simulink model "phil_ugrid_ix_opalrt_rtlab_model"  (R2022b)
settings: Solver=ode3  StartTime=0.0  StopTime=inf  FixedStep=Ts  RelTol=1e-3
PostLoadFcn:
  | phil_ugrid_ix_opalrt_rtlab_param;
InitFcn:
  | phil_ugrid_ix_opalrt_rtlab_param;
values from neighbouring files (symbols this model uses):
  GridFreq = 50    [phil_ugrid_ix_opalrt_rtlab_param.m]
  KiIg = 1/Ti2*1/5    (= 165)    [phil_ugrid_ix_opalrt_rtlab_param.m]
  KpIg = Tn2/Ti2*1/3    (= 18.3333333333)    [phil_ugrid_ix_opalrt_rtlab_param.m]
  Lg = 2.2e-3    (= 0.0022)    [phil_ugrid_ix_opalrt_rtlab_param.m]
  PLL_BW = 30    [phil_ugrid_ix_opalrt_rtlab_param.m]
  PLL_FREQ = 50    [phil_ugrid_ix_opalrt_rtlab_param.m]
  PLL_zeta = 1/sqrt(2)    [phil_ugrid_ix_opalrt_rtlab_param.m]
undefined symbols (not defined in the file or in its folder): af15, arm1_g1, Boost2lvl_SFun, boost_I, boost_V, C, c62c8459, DB, DiscIntNeverNeededParam, EFPGASIMConfig, eHSBuildReport, eHSx64_Gen4_Machines_IOConfig1, EX, fault_sw, LABv2024, logs, matlab, Min, models, ns, OPAL, phil_ugrid_ix_opalrt_rtlab, phil_ugrid_ix_opalrt_rtlab_ehs, phil_ugrid_ix_opalrt_rtlab_model, phil_ugrid_ix_opalrt_rtlab_param, RT, Step, TE0741_4, Time, Users, v1, vin, vsrc1, vsrc2, vsrc3
libraries: simulink x6, opal_lib x3, rtlab x2, slpidlib x2, rtio_opalrt_common x1, ehsSchematicEditorSourceLib x1

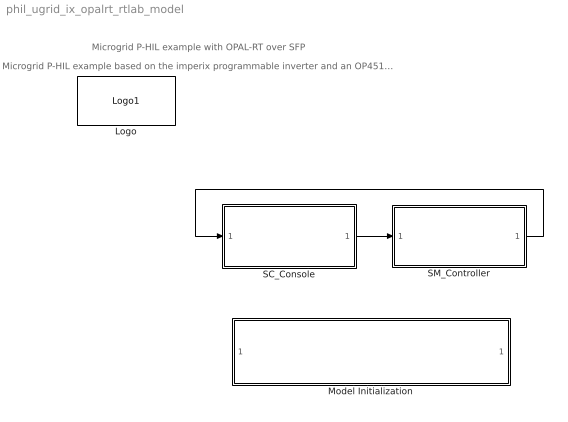
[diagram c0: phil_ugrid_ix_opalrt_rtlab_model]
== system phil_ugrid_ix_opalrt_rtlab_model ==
  note: Microgrid P-HIL example based on the imperix programmable inverter and an OP4510 from OPAL-RT.
  note: Microgrid P-HIL example with OPAL-RT over SFP
  Logo : opal_lib/Logo1  vide=[]
  Model Initialization : Subsystem  mask(Model Functions){InitFcnX=phil_ugrid_ix_opalrt_rtlab_param;, prel=off, posl=on, inif=on, strf=off}
      mask prompts: InitFcnX "Initialisation"; prel "Preload Function"; posl "PostLoad Function"; inif "InitFcn"; strf "StartFcn"
      mask init:
      | currentBlock = gcb;
      | root = bdroot(currentBlock);
      | 
      | if ~strcmp(get_param(root,'BlockDiagramType'),'library')
      |     if prel==1
      |         set_param(root, 'PreLoadFcn', InitFcnX);
      |     else
      |         set_param(root, 'PreLoadFcn', '');
      |     end
      |     if inif==1
      |         set_param(root, 'InitFcn', InitFcnX);
      |     else
      |         set_param(root, 'InitFcn', '');
      |     end
      |     if strf==1
      |         set_param(root, 'StartFcn', InitFcnX);
      |     else
      |         set_param(root, 'StartFcn', '');
      |     end
      |     if posl==1
      |         set_param(root, 'PostLoadFcn', InitFcnX);
      |     else
      |         set_param(root, 'PostLoadFcn', '');
      |     end
      | end
      | 
      | pos = get_param(currentBlock, 'Position');
      | width = pos(3) - pos(1); height = pos(4) - pos(2);
      | txt = [ upper(root) '\n' '- InitFcn. . . . . '  get_param(root, 'InitFcn') ];
  SC_Console : Subsystem
  SM_Controller : Subsystem
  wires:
  SC_Console/1(to_eHS) -> SM_Controller/1(to_eHS)
  SM_Controller/1(from_eHS) -> SC_Console/1(from_eHS)

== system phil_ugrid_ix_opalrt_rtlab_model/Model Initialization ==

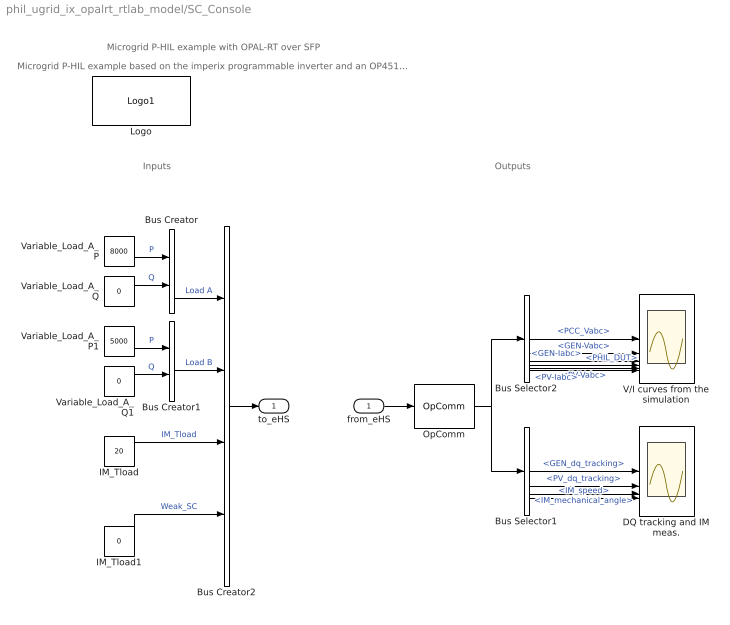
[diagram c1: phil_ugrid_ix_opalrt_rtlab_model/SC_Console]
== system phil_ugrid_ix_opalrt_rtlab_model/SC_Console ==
  note: Inputs
  note: Outputs
  note: Microgrid P-HIL example based on the imperix programmable inverter and an OP4510 from OPAL-RT.
  note: Microgrid P-HIL example with OPAL-RT over SFP
  from_eHS : Inport  OutDataTypeStr=double
  Bus Creator : BusCreator  Inputs=2
  Bus Creator1 : BusCreator  Inputs=2
  Bus Creator2 : BusCreator  Inputs=4
  Bus Selector1 : BusSelector  OutputSignals=signal2.GEN_dq_tracking,signal2.PV_dq_tracking,signal1.IM.IM_mechanical_angle,signal1.IM.IM_speed
  Bus Selector2 : BusSelector  OutputSignals=signal1.PCC_Vabc,signal1.GEN-Vabc,signal1.GEN-Iabc,signal1.PHIL_DUT,signal1.PV-Vabc,signal1.PV-Iabc
  DQ tracking and IM meas. : Scope  NumInputPorts=4
  IM_Tload : Constant  Value=20
  IM_Tload1 : Constant  Value=0
  Logo : opal_lib/Logo1  vide=[]
  OpComm : rtlab/OpComm  nbport=1  groupe_acq=1  subsys_rate=0  st=0  Synchronization=off  Interpolation=off  Threshold=1.0  Missed_Data=off  Sim_Time=off  Samples=off  dynSigOut=off  from_console=0  warning_done=off  writeOpCommFile=off
  V/I curves from the simulation : Scope  NumInputPorts=6
  Variable_Load_A_P : Constant  Value=8000
  Variable_Load_A_P1 : Constant  Value=5000
  Variable_Load_A_Q : Constant  Value=0
  Variable_Load_A_Q1 : Constant  Value=0
  to_eHS : Outport  VectorParamsAs1DForOutWhenUnconnected=off
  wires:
  from_eHS/1 -> OpComm/1
  Bus Creator2/1 -> to_eHS/1
  OpComm/1 -> Bus Selector1/1, Bus Selector2/1
  Variable_Load_A_P/1 -> Bus Creator/1  "P"
  Variable_Load_A_Q/1 -> Bus Creator/2  "Q"
  Variable_Load_A_P1/1 -> Bus Creator1/1  "P"
  Variable_Load_A_Q1/1 -> Bus Creator1/2  "Q"
  Bus Creator/1 -> Bus Creator2/1  "Load A"
  Bus Creator1/1 -> Bus Creator2/2  "Load B"
  IM_Tload/1 -> Bus Creator2/3  "IM_Tload"
  Bus Selector2/1 -> V/I curves from the simulation/1  "<PCC_Vabc>"
  Bus Selector2/2 -> V/I curves from the simulation/2  "<GEN-Vabc>"
  Bus Selector2/3 -> V/I curves from the simulation/3  "<GEN-Iabc>"
  Bus Selector2/4 -> V/I curves from the simulation/4  "<PHIL_DUT>"
  Bus Selector2/5 -> V/I curves from the simulation/5  "<PV-Vabc>"
  Bus Selector2/6 -> V/I curves from the simulation/6  "<PV-Iabc>"
  Bus Selector1/1 -> DQ tracking and IM meas./1  "<GEN_dq_tracking>"
  Bus Selector1/2 -> DQ tracking and IM meas./2  "<PV_dq_tracking>"
  Bus Selector1/3 -> DQ tracking and IM meas./3  "<IM_mechanical_angle>"
  Bus Selector1/4 -> DQ tracking and IM meas./4  "<IM_speed>"
  IM_Tload1/1 -> Bus Creator2/4  "Weak_SC"

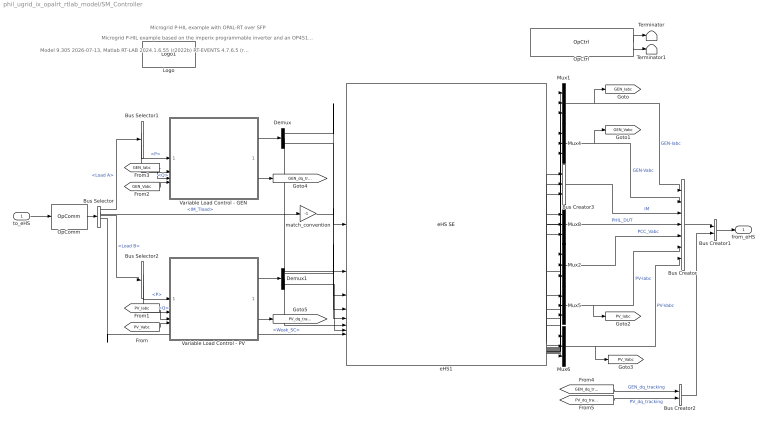
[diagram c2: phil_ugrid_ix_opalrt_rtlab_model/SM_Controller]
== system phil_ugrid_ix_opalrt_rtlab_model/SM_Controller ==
  note: Model 9.305 2026-07-13, Matlab RT-LAB 2024.1.6.55 (r2022b) RT-EVENTS 4.7.6.5 (r2022b.x) eFPGAsim () &copy; 2026 Opal-RT Technologies Inc.
  note: Microgrid P-HIL example with OPAL-RT over SFP
  note: Microgrid P-HIL example based on the imperix programmable inverter and an OP4510 from OPAL-RT.
  to_eHS : Inport
  Bus Creator : BusCreator  Inputs=7
  Bus Creator1 : BusCreator  Inputs=2
  Bus Creator2 : BusCreator  Inputs=2
  Bus Creator3 : BusCreator  Inputs=3
  Bus Selector : BusSelector  OutputSignals=Load A,IM_Tload,Load B,Weak_SC
  Bus Selector1 : BusSelector  OutputSignals=P,Q
  Bus Selector2 : BusSelector  OutputSignals=P,Q
  Demux : Demux  Outputs=3
  Demux1 : Demux  Outputs=3
  Logo : opal_lib/Logo1  vide=[]
  Mux{1..2,4..6,8} (6 alike) : Mux  Inputs=3
  OpComm : rtlab/OpComm  nbport=1  groupe_acq=1  subsys_rate=0  st=0  Synchronization=on  Interpolation=on  Threshold=1.0  Missed_Data=off  Sim_Time=off  Samples=off  dynSigOut=off  from_console=1  warning_done=off  writeOpCommFile=off
  OpCtrl : rtio_opalrt_common/OpCtrl  CtrlName='OpCtrl'  boardid=0  BitstreamFilename=TE0741_4-EX-0001-3_11_2_12-eHSx64_Gen4_Machines_IOConfig1-DB-4A.bin  numconfig=-1  mode=Master  externalClock=off  decimRtsi=0  calibIO=off  SampleTime=0  loadinport=-1  BoardType=TE0741  SecondaryPresent=off  sync_type=Audio  scope_enable=off  fsdFileName=TE0741_4-EX-0001-3_11_2_12-eHSx64_Gen4_Machines_IOConfig1-DB-4A.fsd  mismatch_disable=on
  Terminator : Terminator
  Terminator1 : Terminator
  Variable Load Control - GEN : Subsystem
  Variable Load Control - PV : Subsystem
  eHS1 : ehsSchematicEditorSourceLib/eHS SE  modelName=Boost2lvl_SFun - v1  modelUuid=c62c8459-3f79-48c0-af15-759a73c628dc  modelDisplayName=Boost2lvl_SFun  lastLoadedModelText=Circuit loaded on 09-Oct-2024 14:20:43  lastLoadedModelName=Boost2lvl_SFun - v1  lastLoadedModelUuid=c62c8459-3f79-48c0-af15-759a73c628dc  lastLoadedModelDisplayName=Boost2lvl_SFun - v1  triggerUpdate=off  timeStepInfo=Time Step: 230 ns (Min: 230 ns)  inputPins=arm1_g1,fault_sw,vin,vsrc1,vsrc2,vsrc3  outputPins=2Lvl_Ia,2Lvl_Ib,2Lvl_Ic,2Lvl_Va,2Lvl_Vb,2Lvl_Vc,boost_I,boost_V  loadPassed=1  firmwareName=TE0741_4-EX-0001-3_11_2_12-eHSx64_Gen4_Machines_IOConfig1-DB-4A.bin  driverType=SFUN  ehsEffectiveLicense=x128  migrated=on  opCtrlName='OpCtrl'  autoConfigureFirmware=on  ehsFileName=phil_ugrid_ix_opalrt_rtlab_ehs.ehs3  buildReportFile=C:\Users\matlab\OPAL-RT\RT-LABv2024.1_Workspace2\phil_ugrid_ix_opalrt_rtlab\models\phil_ugrid_ix_opalrt_rtlab_model\EFPGASIMConfig\logs\phil_ugrid_ix_opalrt_rtlab_ehs\logs\eHSBuildReport.txt  displayBlockInfos=|
      | x32
      | Time Step: 355 ns (Min: 355 ns)
  match_convention : Gain  Gain=-1
  from_eHS : Outport  VectorParamsAs1DForOutWhenUnconnected=off
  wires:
  to_eHS/1 -> OpComm/1
  OpComm/1 -> Bus Selector/1
  OpCtrl/1 -> Terminator/1
  OpCtrl/2 -> Terminator1/1
  Mux2/1 -> Bus Creator/5  "PCC_Vabc"
  Bus Selector1/1 -> Variable Load Control - GEN/1(P)  "<P>"
  Bus Selector1/2 -> Variable Load Control - GEN/2(Q)  "<Q>"
  Bus Selector/1 -> Bus Selector1/1  "<Load A>"
  Variable Load Control - GEN/1(Vabc) -> Demux/1
  Demux/2 -> eHS1/2
  Demux/1 -> eHS1/1
  Demux/3 -> eHS1/3
  Variable Load Control - PV/1(Vabc) -> Demux1/1
  Demux1/2 -> eHS1/6
  Demux1/3 -> eHS1/7
  Bus Selector/3 -> Bus Selector2/1  "<Load B>"
  Bus Selector2/2 -> Variable Load Control - PV/2(Q)  "<Q>"
  Bus Selector2/1 -> Variable Load Control - PV/1(P)  "<P>"
  eHS1/1 -> Mux1/1
  eHS1/2 -> Mux1/2
  eHS1/3 -> Mux1/3
  eHS1/4 -> Mux4/1
  eHS1/5 -> Mux4/2
  eHS1/6 -> Mux4/3
  Mux1/1 -> Bus Creator/1, [GEN_Iabc]  "GEN-Iabc"
  Mux4/1 -> Bus Creator/2, [GEN_Vabc]  "GEN-Vabc"
  Mux5/1 -> Bus Creator/6, [PV_Iabc]  "PV-Iabc"
  Mux6/1 -> Bus Creator/7, [PV_Vabc]  "PV-Vabc"
  [PV_Vabc] -> Variable Load Control - PV/4(vabc)
  [PV_Iabc] -> Variable Load Control - PV/3(iabc)
  [GEN_Vabc] -> Variable Load Control - GEN/4(vabc)
  [GEN_Iabc] -> Variable Load Control - GEN/3(iabc)
  Mux8/1 -> Bus Creator/4  "PHIL_DUT"
  Bus Selector/2 -> match_convention/1  "<IM_Tload>"
  eHS1/10 -> Mux8/1
  eHS1/11 -> Mux8/2
  eHS1/12 -> Mux8/3
  eHS1/13 -> Mux2/1
  eHS1/14 -> Mux2/2
  eHS1/15 -> Mux2/3
  eHS1/16 -> Mux5/1
  eHS1/17 -> Mux5/2
  eHS1/18 -> Mux5/3
  eHS1/19 -> Mux6/1
  eHS1/20 -> Mux6/2
  eHS1/21 -> Mux6/3
  Bus Creator3/1 -> Bus Creator/3  "IM"
  eHS1/7 -> Bus Creator3/1
  eHS1/9 -> Bus Creator3/3
  Bus Creator1/1 -> from_eHS/1
  Bus Creator/1 -> Bus Creator1/1
  Bus Creator2/1 -> Bus Creator1/2
  Variable Load Control - GEN/2(dq_tracking) -> [GEN_dq_tracking]
  [GEN_dq_tracking] -> Bus Creator2/1  "GEN_dq_tracking"
  Variable Load Control - PV/2(dq_tracking) -> [PV_dq_tracking]
  [PV_dq_tracking] -> Bus Creator2/2  "PV_dq_tracking"
  Demux1/1 -> eHS1/5
  eHS1/8 -> Bus Creator3/2
  Bus Selector/4 -> eHS1/8  "<Weak_SC>"
  match_convention/1 -> eHS1/4

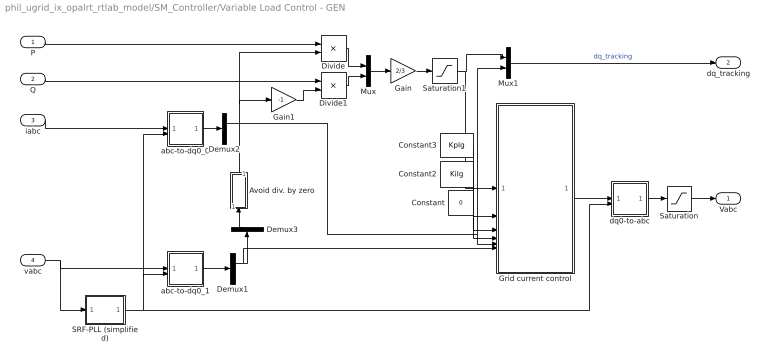
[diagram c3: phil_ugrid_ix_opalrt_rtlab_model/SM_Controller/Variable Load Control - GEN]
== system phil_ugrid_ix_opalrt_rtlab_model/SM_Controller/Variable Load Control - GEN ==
  P : Inport
  Q : Inport  Port=2
  iabc : Inport  Port=3
  vabc : Inport  Port=4
  Avoid div. by zero : Subsystem
  Constant : Constant  Value=0  OutDataTypeStr=double
  Constant2 : Constant  Value=KiIg  OutDataTypeStr=double
  Constant3 : Constant  Value=KpIg  OutDataTypeStr=double
  Demux1 : Demux  Outputs=[2 1]
  Demux2 : Demux  Outputs=[2 1]
  Demux3 : Demux  Outputs=2
  Divide : Product  Inputs=*/
  Divide1 : Product  Inputs=*/
  Gain : Gain  Gain=2/3
  Gain1 : Gain  Gain=-1
  Grid current control : Subsystem
  Mux : Mux  Inputs=2
  Mux1 : Mux  Inputs=2
  SRF-PLL (simplified) : Subsystem
  Saturation : Saturate  UpperLimit=400  LowerLimit=-400
  Saturation1 : Saturate  UpperLimit=50  LowerLimit=-50
  abc-to-dq0_0 : Subsystem
  abc-to-dq0_1 : Subsystem
  dq0-to-abc : Subsystem
  Vabc : Outport
  dq_tracking : Outport  Port=2
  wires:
  Demux3/1 -> Avoid div. by zero/1(In)
  Mux1/1 -> dq_tracking/1  "dq_tracking"
  Divide/1 -> Mux/1
  Divide1/1 -> Mux/2
  Mux/1 -> Gain/1
  Gain1/1 -> Divide1/2
  abc-to-dq0_0/1(dq0) -> Demux2/1
  iabc/1 -> abc-to-dq0_0/1(abc)
  Avoid div. by zero/1(Out) -> Divide/2, Gain1/1
  Gain/1 -> Saturation1/1
  abc-to-dq0_1/1(dq0) -> Demux1/1
  P/1 -> Divide/1
  Q/1 -> Divide1/1
  vabc/1 -> abc-to-dq0_1/1(abc), SRF-PLL (simplified)/1(Vg)
  SRF-PLL (simplified)/1(θ) -> dq0-to-abc/2(wt), abc-to-dq0_0/2(wt), abc-to-dq0_1/2(wt)
  Constant2/1 -> Grid current control/3(Ki_Ig)
  Demux2/1 -> Mux1/2, Grid current control/5(Ig_dq)
  Demux1/1 -> Grid current control/6(Vg_dq), Demux3/1
  Constant/1 -> Grid current control/4(reset)
  Constant3/1 -> Grid current control/2(Kp_Ig)
  Saturation1/1 -> Grid current control/1(Ig_dq_ref), Mux1/1
  dq0-to-abc/1(abc) -> Saturation/1
  Grid current control/1(Eg_dq0*) -> dq0-to-abc/1(dq0)
  Saturation/1 -> Vabc/1

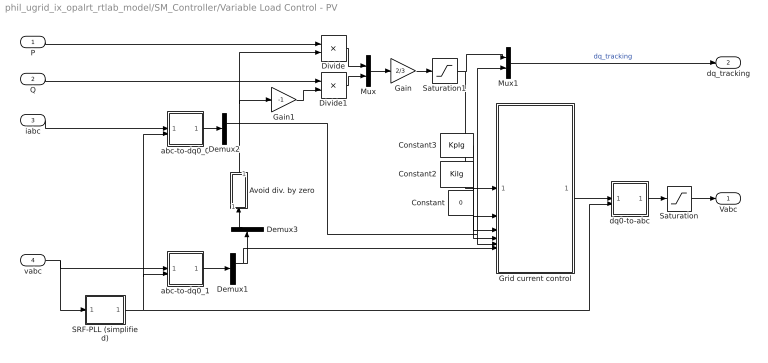
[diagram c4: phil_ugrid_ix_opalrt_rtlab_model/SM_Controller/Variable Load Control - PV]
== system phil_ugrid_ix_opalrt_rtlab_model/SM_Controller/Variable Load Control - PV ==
  P : Inport
  Q : Inport  Port=2
  iabc : Inport  Port=3
  vabc : Inport  Port=4
  Avoid div. by zero : Subsystem
  Constant : Constant  Value=0  OutDataTypeStr=double
  Constant2 : Constant  Value=KiIg  OutDataTypeStr=double
  Constant3 : Constant  Value=KpIg  OutDataTypeStr=double
  Demux1 : Demux  Outputs=[2 1]
  Demux2 : Demux  Outputs=[2 1]
  Demux3 : Demux  Outputs=2
  Divide : Product  Inputs=*/
  Divide1 : Product  Inputs=*/
  Gain : Gain  Gain=2/3
  Gain1 : Gain  Gain=-1
  Grid current control : Subsystem
  Mux : Mux  Inputs=2
  Mux1 : Mux  Inputs=2
  SRF-PLL (simplified) : Subsystem
  Saturation : Saturate  UpperLimit=400  LowerLimit=-400
  Saturation1 : Saturate  UpperLimit=50  LowerLimit=-50
  abc-to-dq0_0 : Subsystem
  abc-to-dq0_1 : Subsystem
  dq0-to-abc : Subsystem
  Vabc : Outport
  dq_tracking : Outport  Port=2
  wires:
  Saturation/1 -> Vabc/1
  Grid current control/1(Eg_dq0*) -> dq0-to-abc/1(dq0)
  dq0-to-abc/1(abc) -> Saturation/1
  Saturation1/1 -> Mux1/1, Grid current control/1(Ig_dq_ref)
  Constant3/1 -> Grid current control/2(Kp_Ig)
  Constant/1 -> Grid current control/4(reset)
  Demux1/1 -> Demux3/1, Grid current control/6(Vg_dq)
  Demux2/1 -> Grid current control/5(Ig_dq), Mux1/2
  Constant2/1 -> Grid current control/3(Ki_Ig)
  SRF-PLL (simplified)/1(θ) -> abc-to-dq0_1/2(wt), abc-to-dq0_0/2(wt), dq0-to-abc/2(wt)
  vabc/1 -> SRF-PLL (simplified)/1(Vg), abc-to-dq0_1/1(abc)
  Q/1 -> Divide1/1
  P/1 -> Divide/1
  abc-to-dq0_1/1(dq0) -> Demux1/1
  Gain/1 -> Saturation1/1
  Avoid div. by zero/1(Out) -> Gain1/1, Divide/2
  iabc/1 -> abc-to-dq0_0/1(abc)
  abc-to-dq0_0/1(dq0) -> Demux2/1
  Gain1/1 -> Divide1/2
  Mux/1 -> Gain/1
  Divide1/1 -> Mux/2
  Divide/1 -> Mux/1
  Mux1/1 -> dq_tracking/1  "dq_tracking"
  Demux3/1 -> Avoid div. by zero/1(In)

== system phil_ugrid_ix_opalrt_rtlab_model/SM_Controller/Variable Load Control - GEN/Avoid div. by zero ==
  In : Inport
  Abs : Abs
  Compare To Constant : simulink/Logic and Bit Operations/Compare To Constant  relop=>=  const=1e-9  OutDataTypeStr=boolean
  Constant4 : Constant  Value=0.001  OutDataTypeStr=single
  Switch : Switch  Criteria=u2 > Threshold
  Out : Outport
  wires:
  Switch/1 -> Out/1
  Compare To Constant/1 -> Switch/2
  Abs/1 -> Compare To Constant/1
  In/1 -> Switch/1, Abs/1
  Constant4/1 -> Switch/3

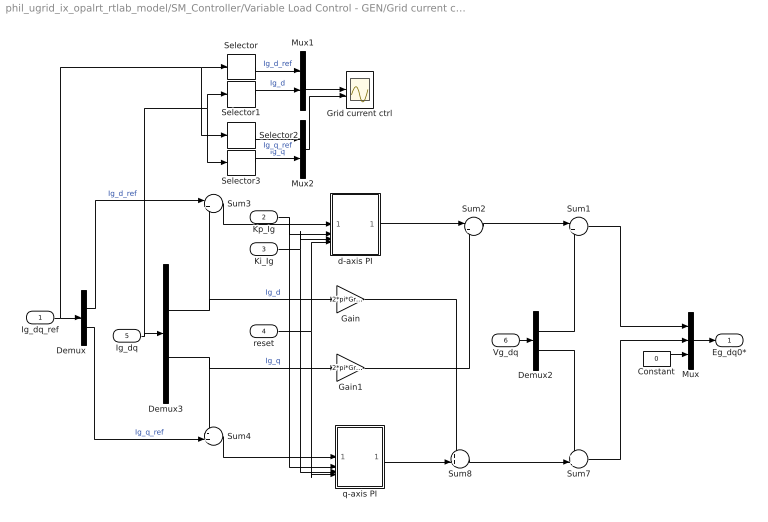
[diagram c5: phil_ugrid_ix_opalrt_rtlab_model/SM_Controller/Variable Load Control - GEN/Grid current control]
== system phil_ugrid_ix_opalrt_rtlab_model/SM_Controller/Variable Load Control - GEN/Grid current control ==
  Ig_dq_ref : Inport
  Kp_Ig : Inport  Port=2
  Ki_Ig : Inport  Port=3
  reset : Inport  Port=4
  Ig_dq : Inport  Port=5
  Vg_dq : Inport  Port=6
  Constant : Constant  Value=0  OutDataTypeStr=double
  Demux : Demux  Outputs=2
  Demux2 : Demux  Outputs=2
  Demux3 : Demux  Outputs=2
  Gain : Gain  Gain=2*pi*GridFreq*Lg
  Gain1 : Gain  Gain=2*pi*GridFreq*Lg
  Grid current ctrl : Scope  NumInputPorts=2
  Mux : Mux  Inputs=3
  Mux1 : Mux  Inputs=2
  Mux2 : Mux  Inputs=2
  Selector : Selector  InputPortWidth=2  IndexOptions=Index vector (dialog)  Indices=[1]  OutputSizes=1
  Selector1 : Selector  InputPortWidth=2  IndexOptions=Index vector (dialog)  Indices=[1]  OutputSizes=1
  Selector2 : Selector  InputPortWidth=2  IndexOptions=Index vector (dialog)  Indices=[2]  OutputSizes=1
  Selector3 : Selector  InputPortWidth=2  IndexOptions=Index vector (dialog)  Indices=[2]  OutputSizes=1
  Sum1 : Sum  Inputs=|++
  Sum2 : Sum  Inputs=|+-
  Sum3 : Sum  Inputs=|+-
  Sum4 : Sum  Inputs=-+|
  Sum7 : Sum  Inputs=++|
  Sum8 : Sum  Inputs=++|
  d-axis PI : Subsystem
  q-axis PI : Subsystem
  Eg_dq0* : Outport
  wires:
  Gain/1 -> Sum8/1
  Gain1/1 -> Sum2/2
  Mux2/1 -> Grid current ctrl/2
  Mux1/1 -> Grid current ctrl/1
  Selector3/1 -> Mux2/2  "Ig_q"
  Selector2/1 -> Mux2/1  "Ig_q_ref"
  Selector/1 -> Mux1/1  "Ig_d_ref"
  Selector1/1 -> Mux1/2  "Ig_d"
  Ig_dq_ref/1 -> Demux/1, Selector/1, Selector2/1
  Sum1/1 -> Mux/1
  Sum7/1 -> Mux/2
  d-axis PI/1(y) -> Sum2/1
  q-axis PI/1(y) -> Sum8/2
  Ig_dq/1 -> Demux3/1, Selector1/1, Selector3/1
  Demux/1 -> Sum3/1  "Ig_d_ref"
  Demux/2 -> Sum4/2  "Ig_q_ref"
  Demux3/1 -> Sum3/2, Gain/1  "Ig_d"
  Demux3/2 -> Sum4/1, Gain1/1  "Ig_q"
  Demux2/2 -> Sum7/1
  Vg_dq/1 -> Demux2/1
  Mux/1 -> Eg_dq0*/1
  Sum2/1 -> Sum1/1
  Sum8/1 -> Sum7/2
  Constant/1 -> Mux/3
  reset/1 -> q-axis PI/4(reset), d-axis PI/4(reset)
  Ki_Ig/1 -> q-axis PI/3(Ki), d-axis PI/3(Ki)
  Kp_Ig/1 -> q-axis PI/2(Kp), d-axis PI/2(Kp)
  Sum3/1 -> d-axis PI/1(e)
  Sum4/1 -> q-axis PI/1(e)
  Demux2/1 -> Sum1/2

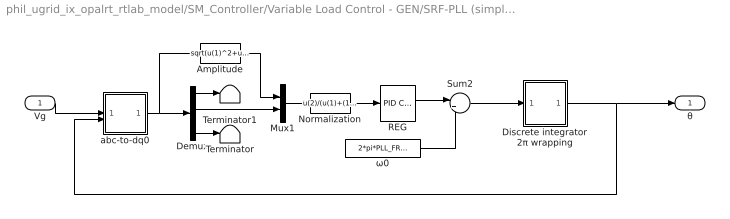
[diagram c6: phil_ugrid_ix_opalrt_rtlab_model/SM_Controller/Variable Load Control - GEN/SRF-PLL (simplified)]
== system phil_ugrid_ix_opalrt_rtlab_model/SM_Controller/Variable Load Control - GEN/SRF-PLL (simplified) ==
  Vg : Inport
  Amplitude : Fcn  Expr=sqrt(u(1)^2+u(2)^2)
  Demux : Demux  Outputs=3
  Discrete integrator 2π wrapping : Subsystem
  Mux1 : Mux  Inputs=2
  Normalization : Fcn  Expr=u(2)/(u(1)+(1e-6)*(u(1)==0))
  REG : slpidlib/PID Controller  Controller=PI  Form=Parallel  TimeDomain=Discrete-time  UseExternalTs=off  SampleTime=-1  IntegratorMethod=Trapezoidal  FilterMethod=Forward Euler  ControllerParametersSource=internal  P=2*2*pi*PLL_BW*PLL_zeta  I=PLL_BW*PLL_BW*4*pi*pi  UseKiTs=off  D=0  N=100  UseFilter=on  TunerSelectOption=Transfer Function Based (PID Tuner App)  InitialConditionSource=internal  InitialConditionForIntegrator=0  InitialConditionForFilter=0  DifferentiatorICPrevScaledInput=0  ExternalReset=none  TrackingMode=off  Kt=1  LimitOutput=off  SatLimitsSource=internal  UpperSaturationLimit=inf  LowerSaturationLimit=-inf  LinearizeAsGain=on  AntiWindupMode=none  Kb=1  LimitIntegrator=off  UpperIntegratorSaturationLimit=inf  LowerIntegratorSaturationLimit=-inf  POutMin=[]  POutMax=[]  IOutMin=[]  IOutMax=[]  DOutMin=[]  DOutMax=[]  NOutMin=[]  NOutMax=[]  SumOutMin=[]  SumOutMax=[]  SaturationOutMin=[]  SaturationOutMax=[]  PParamMin=[]  PParamMax=[]  IParamMin=[]  IParamMax=[]  DParamMin=[]  DParamMax=[]  NParamMin=[]  NParamMax=[]  KbParamMin=[]  KbParamMax=[]  KtParamMin=[]  KtParamMax=[]  KbOutMin=[]  KbOutMax=[]  KtOutMin=[]  KtOutMax=[]  IntegratorOutMin=[]  IntegratorOutMax=[]  FilterOutMin=[]  FilterOutMax=[]  SumI1OutMin=[]  SumI1OutMax=[]  SumI2OutMin=[]  SumI2OutMax=[]  SumI3OutMin=[]  SumI3OutMax=[]  SumI4OutMin=[]  SumI4OutMax=[]  SumDOutMin=[]  SumDOutMax=[]  DifferentiatorOutMin=[]  DifferentiatorOutMax=[]  FilterDiffOutCoefMin=[]  FilterDiffOutCoefMax=[]  ReciprocalOutMin=[]  ReciprocalOutMax=[]  SumDenOutMin=[]  SumDenOutMax=[]  SumNumOutMin=[]  SumNumOutMax=[]  DivideOutMin=[]  DivideOutMax=[]  UdiffTsProdOutMin=[]  UdiffTsProdOutMax=[]  NTsProdOutMin=[]  NTsProdOutMax=[]  UintegralTsProdOutMin=[]  UintegralTsProdOutMax=[]  UngainTsProdOutMin=[]  UngainTsProdOutMax=[]  ClampingZeroOutDataTypeStr=Inherit: Inherit via back propagation  ClampingZeroOutMin=[]  ClampingZeroOutMax=[]  FilterDenConstantOutDataTypeStr=Inherit: Inherit via back propagation  FilterDenConstantOutMin=[]  FilterDenConstantOutMax=[]  PCopyOutDataTypeStr=Inherit: Inherit via back propagation  PCopyOutMin=[]  PCopyOutMax=[]  NCopyOutDataTypeStr=Inherit: Inherit via back propagation  NCopyOutMin=[]  NCopyOutMax=[]  IntegratorContinuousStateAttributes=''  IntegratorStateMustResolveToSignalObject=off  IntegratorRTWStateStorageClass=Auto  FilterContinuousStateAttributes=''  FilterStateMustResolveToSignalObject=off  FilterRTWStateStorageClass=Auto  ParallelPVariant=InternalParameters  IdealPVariant=Disabled  IVariant=InternalParameters  DVariant=Disabled  IntegratorVariant=Discrete  SatVariant=Disabled  AWVariant=Passthrough  PCopyVariant=Disabled  TRVariant=Disabled  FdbkBlocksVariant=Forward  IdealPFdbkVariant=Disabled  SatFdbkVariant=Disabled  DerivativeFilterVariant=Disabled  NVariant=Disabled  NCopyVariant=Disabled_SignalSpec  FilterICVariant=Disabled  IntegratorICVariant=InternalICs  ExternalResetVariant=Disabled  TRSumVariant=Passthrough  SumFdbkVariant=Disabled  SumVariant=Sum_PI  TsampFilterVariant=InternalTs  TsampNgainVariant=Passthrough  TsampIntegralVariant=Passthrough  ExternalSaturationOutDataTypeStr=Inherit: Same as second input
  Sum2 : Sum  Inputs=|++
  Terminator : Terminator
  Terminator1 : Terminator
  abc-to-dq0 : Subsystem
  ω0 : Constant  Value=2*pi*PLL_FREQ  OutDataTypeStr=double
  θ : Outport  OutDataTypeStr=double
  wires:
  Demux/2 -> Mux1/2
  Demux/1 -> Terminator1/1
  Normalization/1 -> REG/1
  Mux1/1 -> Normalization/1
  REG/1 -> Sum2/1
  Vg/1 -> abc-to-dq0/1(abc)
  Discrete integrator 2π wrapping/1(θ) -> θ/1, abc-to-dq0/2(wt)
  Amplitude/1 -> Mux1/1
  abc-to-dq0/1(dq0) -> Amplitude/1, Demux/1
  Demux/3 -> Terminator/1
  ω0/1 -> Sum2/2
  Sum2/1 -> Discrete integrator 2π wrapping/1(ω)

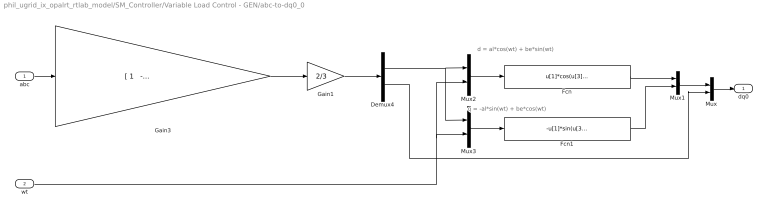
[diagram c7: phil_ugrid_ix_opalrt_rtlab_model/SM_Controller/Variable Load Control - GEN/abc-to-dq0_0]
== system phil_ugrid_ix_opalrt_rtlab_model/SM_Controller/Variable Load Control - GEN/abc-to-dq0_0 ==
  note: q = -al*sin(wt) + be*cos(wt)
  note: d = al*cos(wt) + be*sin(wt)
  abc : Inport  PortDimensions=3
  wt : Inport  Port=2  PortDimensions=1
  Demux4 : Demux  Outputs=[2 1]
  Fcn : Fcn  Expr=u[1]*cos(u[3]) + u[2]*sin(u[3])
  Fcn1 : Fcn  Expr=-u[1]*sin(u[3]) + u[2]*cos(u[3])
  Gain1 : Gain  Gain=2/3  SaturateOnIntegerOverflow=on
  Gain3 : Gain  Gain="[ 1   -1/2   -1/2; 0   sqrt(3)/2   -sqrt(3)/2; 1/2  1/2  1/2 ]"  Multiplication=Matrix(K*u) (u vector)  SaturateOnIntegerOverflow=on
  Mux : Mux  Inputs=[2 1]
  Mux1 : Mux  Inputs=2
  Mux2 : Mux  Inputs=[2 1]
  Mux3 : Mux  Inputs=[2 1]
  dq0 : Outport
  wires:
  Gain1/1 -> Demux4/1
  abc/1 -> Gain3/1
  Demux4/2 -> Mux/2
  Fcn1/1 -> Mux1/2
  Demux4/1 -> Mux3/1, Mux2/1
  Fcn/1 -> Mux1/1
  Mux2/1 -> Fcn/1
  Mux3/1 -> Fcn1/1
  wt/1 -> Mux2/2, Mux3/2
  Mux/1 -> dq0/1
  Mux1/1 -> Mux/1
  Gain3/1 -> Gain1/1

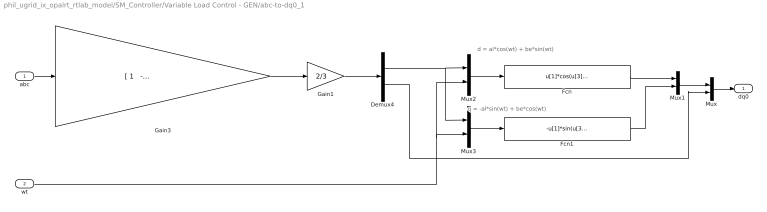
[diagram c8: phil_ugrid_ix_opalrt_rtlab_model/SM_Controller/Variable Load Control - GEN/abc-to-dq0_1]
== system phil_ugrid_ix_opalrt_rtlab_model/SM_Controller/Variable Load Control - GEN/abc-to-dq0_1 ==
  note: d = al*cos(wt) + be*sin(wt)
  note: q = -al*sin(wt) + be*cos(wt)
  abc : Inport  PortDimensions=3
  wt : Inport  Port=2  PortDimensions=1
  Demux4 : Demux  Outputs=[2 1]
  Fcn : Fcn  Expr=u[1]*cos(u[3]) + u[2]*sin(u[3])
  Fcn1 : Fcn  Expr=-u[1]*sin(u[3]) + u[2]*cos(u[3])
  Gain1 : Gain  Gain=2/3  SaturateOnIntegerOverflow=on
  Gain3 : Gain  Gain="[ 1   -1/2   -1/2; 0   sqrt(3)/2   -sqrt(3)/2; 1/2  1/2  1/2 ]"  Multiplication=Matrix(K*u) (u vector)  SaturateOnIntegerOverflow=on
  Mux : Mux  Inputs=[2 1]
  Mux1 : Mux  Inputs=2
  Mux2 : Mux  Inputs=[2 1]
  Mux3 : Mux  Inputs=[2 1]
  dq0 : Outport
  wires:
  Gain3/1 -> Gain1/1
  Mux1/1 -> Mux/1
  Mux/1 -> dq0/1
  wt/1 -> Mux3/2, Mux2/2
  Mux3/1 -> Fcn1/1
  Mux2/1 -> Fcn/1
  Fcn/1 -> Mux1/1
  Demux4/1 -> Mux2/1, Mux3/1
  Fcn1/1 -> Mux1/2
  Demux4/2 -> Mux/2
  abc/1 -> Gain3/1
  Gain1/1 -> Demux4/1

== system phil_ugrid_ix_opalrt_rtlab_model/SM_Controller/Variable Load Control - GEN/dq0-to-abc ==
  dq0 : Inport  PortDimensions=3
  wt : Inport  Port=2  PortDimensions=1
  Demux4 : Demux  Outputs=[2 1]
  Fcn : Fcn  Expr=u[1]*cos(u[3]) - u[2]*sin(u[3])
  Fcn1 : Fcn  Expr=u[1]*sin(u[3]) + u[2]*cos(u[3])
  Gain3 : Gain  Gain="[ 1   0   1; -1/2  sqrt(3)/2   1; -1/2  -sqrt(3)/2  1 ]"  Multiplication=Matrix(K*u) (u vector)  SaturateOnIntegerOverflow=on
  Mux : Mux  Inputs=[2 1]
  Mux1 : Mux  Inputs=2
  Mux2 : Mux  Inputs=[2 1]
  Mux3 : Mux  Inputs=[2 1]
  abc : Outport
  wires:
  Fcn1/1 -> Mux1/2
  Demux4/1 -> Mux2/1, Mux3/1
  wt/1 -> Mux2/2, Mux3/2
  dq0/1 -> Demux4/1
  Gain3/1 -> abc/1
  Fcn/1 -> Mux1/1
  Demux4/2 -> Mux/2
  Mux1/1 -> Mux/1
  Mux/1 -> Gain3/1
  Mux3/1 -> Fcn1/1
  Mux2/1 -> Fcn/1

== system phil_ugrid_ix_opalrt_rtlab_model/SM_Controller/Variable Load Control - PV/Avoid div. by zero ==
  In : Inport
  Abs : Abs
  Compare To Constant : simulink/Logic and Bit Operations/Compare To Constant  relop=>=  const=1e-9  OutDataTypeStr=boolean
  Constant4 : Constant  Value=0.001  OutDataTypeStr=single
  Switch : Switch  Criteria=u2 > Threshold
  Out : Outport
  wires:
  Constant4/1 -> Switch/3
  In/1 -> Abs/1, Switch/1
  Abs/1 -> Compare To Constant/1
  Compare To Constant/1 -> Switch/2
  Switch/1 -> Out/1

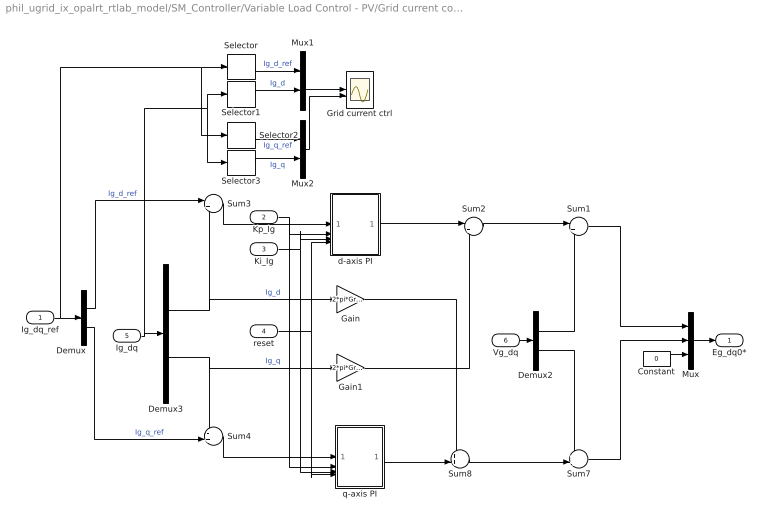
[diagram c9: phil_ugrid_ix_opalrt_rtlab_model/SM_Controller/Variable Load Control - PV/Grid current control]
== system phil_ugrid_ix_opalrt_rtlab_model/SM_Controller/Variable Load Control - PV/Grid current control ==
  Ig_dq_ref : Inport
  Kp_Ig : Inport  Port=2
  Ki_Ig : Inport  Port=3
  reset : Inport  Port=4
  Ig_dq : Inport  Port=5
  Vg_dq : Inport  Port=6
  Constant : Constant  Value=0  OutDataTypeStr=double
  Demux : Demux  Outputs=2
  Demux2 : Demux  Outputs=2
  Demux3 : Demux  Outputs=2
  Gain : Gain  Gain=2*pi*GridFreq*Lg
  Gain1 : Gain  Gain=2*pi*GridFreq*Lg
  Grid current ctrl : Scope  NumInputPorts=2
  Mux : Mux  Inputs=3
  Mux1 : Mux  Inputs=2
  Mux2 : Mux  Inputs=2
  Selector : Selector  InputPortWidth=2  IndexOptions=Index vector (dialog)  Indices=[1]  OutputSizes=1
  Selector1 : Selector  InputPortWidth=2  IndexOptions=Index vector (dialog)  Indices=[1]  OutputSizes=1
  Selector2 : Selector  InputPortWidth=2  IndexOptions=Index vector (dialog)  Indices=[2]  OutputSizes=1
  Selector3 : Selector  InputPortWidth=2  IndexOptions=Index vector (dialog)  Indices=[2]  OutputSizes=1
  Sum1 : Sum  Inputs=|++
  Sum2 : Sum  Inputs=|+-
  Sum3 : Sum  Inputs=|+-
  Sum4 : Sum  Inputs=-+|
  Sum7 : Sum  Inputs=++|
  Sum8 : Sum  Inputs=++|
  d-axis PI : Subsystem
  q-axis PI : Subsystem
  Eg_dq0* : Outport
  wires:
  Demux2/1 -> Sum1/2
  Sum4/1 -> q-axis PI/1(e)
  Sum3/1 -> d-axis PI/1(e)
  Kp_Ig/1 -> d-axis PI/2(Kp), q-axis PI/2(Kp)
  Ki_Ig/1 -> d-axis PI/3(Ki), q-axis PI/3(Ki)
  reset/1 -> d-axis PI/4(reset), q-axis PI/4(reset)
  Constant/1 -> Mux/3
  Sum8/1 -> Sum7/2
  Sum2/1 -> Sum1/1
  Mux/1 -> Eg_dq0*/1
  Vg_dq/1 -> Demux2/1
  Demux2/2 -> Sum7/1
  Demux3/2 -> Gain1/1, Sum4/1  "Ig_q"
  Demux3/1 -> Gain/1, Sum3/2  "Ig_d"
  Demux/2 -> Sum4/2  "Ig_q_ref"
  Demux/1 -> Sum3/1  "Ig_d_ref"
  Ig_dq/1 -> Selector3/1, Selector1/1, Demux3/1
  q-axis PI/1(y) -> Sum8/2
  d-axis PI/1(y) -> Sum2/1
  Sum7/1 -> Mux/2
  Sum1/1 -> Mux/1
  Ig_dq_ref/1 -> Selector2/1, Selector/1, Demux/1
  Selector1/1 -> Mux1/2  "Ig_d"
  Selector/1 -> Mux1/1  "Ig_d_ref"
  Selector2/1 -> Mux2/1  "Ig_q_ref"
  Selector3/1 -> Mux2/2  "Ig_q"
  Mux1/1 -> Grid current ctrl/1
  Mux2/1 -> Grid current ctrl/2
  Gain1/1 -> Sum2/2
  Gain/1 -> Sum8/1

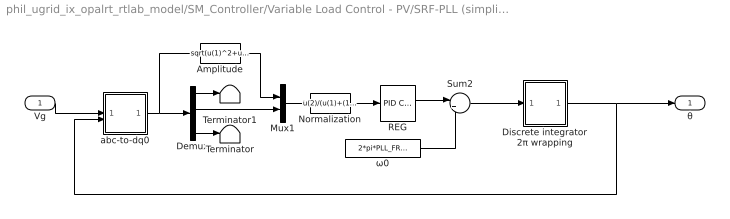
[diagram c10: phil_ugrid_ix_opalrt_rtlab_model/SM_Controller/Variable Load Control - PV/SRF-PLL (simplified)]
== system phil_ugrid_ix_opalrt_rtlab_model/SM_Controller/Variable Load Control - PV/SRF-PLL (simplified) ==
  Vg : Inport
  Amplitude : Fcn  Expr=sqrt(u(1)^2+u(2)^2)
  Demux : Demux  Outputs=3
  Discrete integrator 2π wrapping : Subsystem
  Mux1 : Mux  Inputs=2
  Normalization : Fcn  Expr=u(2)/(u(1)+(1e-6)*(u(1)==0))
  REG : slpidlib/PID Controller  Controller=PI  Form=Parallel  TimeDomain=Discrete-time  UseExternalTs=off  SampleTime=-1  IntegratorMethod=Trapezoidal  FilterMethod=Forward Euler  ControllerParametersSource=internal  P=2*2*pi*PLL_BW*PLL_zeta  I=PLL_BW*PLL_BW*4*pi*pi  UseKiTs=off  D=0  N=100  UseFilter=on  TunerSelectOption=Transfer Function Based (PID Tuner App)  InitialConditionSource=internal  InitialConditionForIntegrator=0  InitialConditionForFilter=0  DifferentiatorICPrevScaledInput=0  ExternalReset=none  TrackingMode=off  Kt=1  LimitOutput=off  SatLimitsSource=internal  UpperSaturationLimit=inf  LowerSaturationLimit=-inf  LinearizeAsGain=on  AntiWindupMode=none  Kb=1  LimitIntegrator=off  UpperIntegratorSaturationLimit=inf  LowerIntegratorSaturationLimit=-inf  POutMin=[]  POutMax=[]  IOutMin=[]  IOutMax=[]  DOutMin=[]  DOutMax=[]  NOutMin=[]  NOutMax=[]  SumOutMin=[]  SumOutMax=[]  SaturationOutMin=[]  SaturationOutMax=[]  PParamMin=[]  PParamMax=[]  IParamMin=[]  IParamMax=[]  DParamMin=[]  DParamMax=[]  NParamMin=[]  NParamMax=[]  KbParamMin=[]  KbParamMax=[]  KtParamMin=[]  KtParamMax=[]  KbOutMin=[]  KbOutMax=[]  KtOutMin=[]  KtOutMax=[]  IntegratorOutMin=[]  IntegratorOutMax=[]  FilterOutMin=[]  FilterOutMax=[]  SumI1OutMin=[]  SumI1OutMax=[]  SumI2OutMin=[]  SumI2OutMax=[]  SumI3OutMin=[]  SumI3OutMax=[]  SumI4OutMin=[]  SumI4OutMax=[]  SumDOutMin=[]  SumDOutMax=[]  DifferentiatorOutMin=[]  DifferentiatorOutMax=[]  FilterDiffOutCoefMin=[]  FilterDiffOutCoefMax=[]  ReciprocalOutMin=[]  ReciprocalOutMax=[]  SumDenOutMin=[]  SumDenOutMax=[]  SumNumOutMin=[]  SumNumOutMax=[]  DivideOutMin=[]  DivideOutMax=[]  UdiffTsProdOutMin=[]  UdiffTsProdOutMax=[]  NTsProdOutMin=[]  NTsProdOutMax=[]  UintegralTsProdOutMin=[]  UintegralTsProdOutMax=[]  UngainTsProdOutMin=[]  UngainTsProdOutMax=[]  ClampingZeroOutDataTypeStr=Inherit: Inherit via back propagation  ClampingZeroOutMin=[]  ClampingZeroOutMax=[]  FilterDenConstantOutDataTypeStr=Inherit: Inherit via back propagation  FilterDenConstantOutMin=[]  FilterDenConstantOutMax=[]  PCopyOutDataTypeStr=Inherit: Inherit via back propagation  PCopyOutMin=[]  PCopyOutMax=[]  NCopyOutDataTypeStr=Inherit: Inherit via back propagation  NCopyOutMin=[]  NCopyOutMax=[]  IntegratorContinuousStateAttributes=''  IntegratorStateMustResolveToSignalObject=off  IntegratorRTWStateStorageClass=Auto  FilterContinuousStateAttributes=''  FilterStateMustResolveToSignalObject=off  FilterRTWStateStorageClass=Auto  ParallelPVariant=InternalParameters  IdealPVariant=Disabled  IVariant=InternalParameters  DVariant=Disabled  IntegratorVariant=Discrete  SatVariant=Disabled  AWVariant=Passthrough  PCopyVariant=Disabled  TRVariant=Disabled  FdbkBlocksVariant=Forward  IdealPFdbkVariant=Disabled  SatFdbkVariant=Disabled  DerivativeFilterVariant=Disabled  NVariant=Disabled  NCopyVariant=Disabled_SignalSpec  FilterICVariant=Disabled  IntegratorICVariant=InternalICs  ExternalResetVariant=Disabled  TRSumVariant=Passthrough  SumFdbkVariant=Disabled  SumVariant=Sum_PI  TsampFilterVariant=InternalTs  TsampNgainVariant=Passthrough  TsampIntegralVariant=Passthrough  ExternalSaturationOutDataTypeStr=Inherit: Same as second input
  Sum2 : Sum  Inputs=|++
  Terminator : Terminator
  Terminator1 : Terminator
  abc-to-dq0 : Subsystem
  ω0 : Constant  Value=2*pi*PLL_FREQ  OutDataTypeStr=double
  θ : Outport  OutDataTypeStr=double
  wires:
  Sum2/1 -> Discrete integrator 2π wrapping/1(ω)
  ω0/1 -> Sum2/2
  Demux/3 -> Terminator/1
  abc-to-dq0/1(dq0) -> Demux/1, Amplitude/1
  Amplitude/1 -> Mux1/1
  Discrete integrator 2π wrapping/1(θ) -> abc-to-dq0/2(wt), θ/1
  Vg/1 -> abc-to-dq0/1(abc)
  REG/1 -> Sum2/1
  Mux1/1 -> Normalization/1
  Normalization/1 -> REG/1
  Demux/1 -> Terminator1/1
  Demux/2 -> Mux1/2

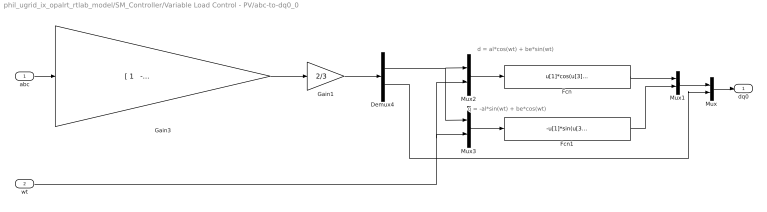
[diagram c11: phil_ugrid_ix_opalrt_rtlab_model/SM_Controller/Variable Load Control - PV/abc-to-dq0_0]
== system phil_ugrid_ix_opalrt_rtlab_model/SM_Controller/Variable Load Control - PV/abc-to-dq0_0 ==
  note: d = al*cos(wt) + be*sin(wt)
  note: q = -al*sin(wt) + be*cos(wt)
  abc : Inport  PortDimensions=3
  wt : Inport  Port=2  PortDimensions=1
  Demux4 : Demux  Outputs=[2 1]
  Fcn : Fcn  Expr=u[1]*cos(u[3]) + u[2]*sin(u[3])
  Fcn1 : Fcn  Expr=-u[1]*sin(u[3]) + u[2]*cos(u[3])
  Gain1 : Gain  Gain=2/3  SaturateOnIntegerOverflow=on
  Gain3 : Gain  Gain="[ 1   -1/2   -1/2; 0   sqrt(3)/2   -sqrt(3)/2; 1/2  1/2  1/2 ]"  Multiplication=Matrix(K*u) (u vector)  SaturateOnIntegerOverflow=on
  Mux : Mux  Inputs=[2 1]
  Mux1 : Mux  Inputs=2
  Mux2 : Mux  Inputs=[2 1]
  Mux3 : Mux  Inputs=[2 1]
  dq0 : Outport
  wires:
  Gain3/1 -> Gain1/1
  Mux1/1 -> Mux/1
  Mux/1 -> dq0/1
  wt/1 -> Mux3/2, Mux2/2
  Mux3/1 -> Fcn1/1
  Mux2/1 -> Fcn/1
  Fcn/1 -> Mux1/1
  Demux4/1 -> Mux2/1, Mux3/1
  Fcn1/1 -> Mux1/2
  Demux4/2 -> Mux/2
  abc/1 -> Gain3/1
  Gain1/1 -> Demux4/1

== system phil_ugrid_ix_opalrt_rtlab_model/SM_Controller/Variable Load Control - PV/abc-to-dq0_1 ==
  note: q = -al*sin(wt) + be*cos(wt)
  note: d = al*cos(wt) + be*sin(wt)
  abc : Inport  PortDimensions=3
  wt : Inport  Port=2  PortDimensions=1
  Demux4 : Demux  Outputs=[2 1]
  Fcn : Fcn  Expr=u[1]*cos(u[3]) + u[2]*sin(u[3])
  Fcn1 : Fcn  Expr=-u[1]*sin(u[3]) + u[2]*cos(u[3])
  Gain1 : Gain  Gain=2/3  SaturateOnIntegerOverflow=on
  Gain3 : Gain  Gain="[ 1   -1/2   -1/2; 0   sqrt(3)/2   -sqrt(3)/2; 1/2  1/2  1/2 ]"  Multiplication=Matrix(K*u) (u vector)  SaturateOnIntegerOverflow=on
  Mux : Mux  Inputs=[2 1]
  Mux1 : Mux  Inputs=2
  Mux2 : Mux  Inputs=[2 1]
  Mux3 : Mux  Inputs=[2 1]
  dq0 : Outport
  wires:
  Gain1/1 -> Demux4/1
  abc/1 -> Gain3/1
  Demux4/2 -> Mux/2
  Fcn1/1 -> Mux1/2
  Demux4/1 -> Mux3/1, Mux2/1
  Fcn/1 -> Mux1/1
  Mux2/1 -> Fcn/1
  Mux3/1 -> Fcn1/1
  wt/1 -> Mux2/2, Mux3/2
  Mux/1 -> dq0/1
  Mux1/1 -> Mux/1
  Gain3/1 -> Gain1/1

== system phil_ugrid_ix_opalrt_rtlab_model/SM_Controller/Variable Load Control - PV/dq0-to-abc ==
  dq0 : Inport  PortDimensions=3
  wt : Inport  Port=2  PortDimensions=1
  Demux4 : Demux  Outputs=[2 1]
  Fcn : Fcn  Expr=u[1]*cos(u[3]) - u[2]*sin(u[3])
  Fcn1 : Fcn  Expr=u[1]*sin(u[3]) + u[2]*cos(u[3])
  Gain3 : Gain  Gain="[ 1   0   1; -1/2  sqrt(3)/2   1; -1/2  -sqrt(3)/2  1 ]"  Multiplication=Matrix(K*u) (u vector)  SaturateOnIntegerOverflow=on
  Mux : Mux  Inputs=[2 1]
  Mux1 : Mux  Inputs=2
  Mux2 : Mux  Inputs=[2 1]
  Mux3 : Mux  Inputs=[2 1]
  abc : Outport
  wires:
  Mux2/1 -> Fcn/1
  Mux3/1 -> Fcn1/1
  Mux/1 -> Gain3/1
  Mux1/1 -> Mux/1
  Demux4/2 -> Mux/2
  Fcn/1 -> Mux1/1
  Gain3/1 -> abc/1
  dq0/1 -> Demux4/1
  wt/1 -> Mux3/2, Mux2/2
  Demux4/1 -> Mux3/1, Mux2/1
  Fcn1/1 -> Mux1/2

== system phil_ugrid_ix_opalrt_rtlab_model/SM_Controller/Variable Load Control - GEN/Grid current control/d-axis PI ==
  e : Inport
  Kp : Inport  Port=2
  Ki : Inport  Port=3
  reset : Inport  Port=4
  IOut : Product  DisableCoverage=on
  Integrator : DiscreteIntegrator  ExternalReset=level  SampleTime=-1  ICPrevOutput=DiscIntNeverNeededParam  ICPrevScaledInput=DiscIntNeverNeededParam
  POut : Product
  Sum1 : Sum  Inputs=|++
  y : Outport  InitialOutput=0
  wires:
  e/1 -> POut/1, IOut/1
  Sum1/1 -> y/1
  Ki/1 -> IOut/2
  Kp/1 -> POut/2
  reset/1 -> Integrator/2
  IOut/1 -> Integrator/1
  POut/1 -> Sum1/2
  Integrator/1 -> Sum1/1

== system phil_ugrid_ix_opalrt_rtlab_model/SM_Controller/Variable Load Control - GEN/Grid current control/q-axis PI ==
  e : Inport
  Kp : Inport  Port=2
  Ki : Inport  Port=3
  reset : Inport  Port=4
  IOut : Product  DisableCoverage=on
  Integrator : DiscreteIntegrator  ExternalReset=level  SampleTime=-1  ICPrevOutput=DiscIntNeverNeededParam  ICPrevScaledInput=DiscIntNeverNeededParam
  POut : Product
  Sum1 : Sum  Inputs=|++
  y : Outport  InitialOutput=0
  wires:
  Integrator/1 -> Sum1/1
  POut/1 -> Sum1/2
  IOut/1 -> Integrator/1
  reset/1 -> Integrator/2
  Kp/1 -> POut/2
  Ki/1 -> IOut/2
  Sum1/1 -> y/1
  e/1 -> IOut/1, POut/1

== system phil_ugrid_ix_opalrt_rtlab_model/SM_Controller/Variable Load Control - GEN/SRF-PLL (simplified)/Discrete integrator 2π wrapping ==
  ω : Inport
  Compare To Constant : simulink/Logic and Bit Operations/Compare To Constant  relop=<  const=0  OutDataTypeStr=boolean
  Compare To Constant1 : simulink/Logic and Bit Operations/Compare To Constant  relop=>=  const=2*pi  OutDataTypeStr=boolean
  Discrete-Time Integrator : DiscreteIntegrator  ExternalReset=sampled level  InitialConditionSource=external  SampleTime=-1  ShowStatePort=on  ICPrevOutput=DiscIntNeverNeededParam  ICPrevScaledInput=DiscIntNeverNeededParam
  Gain : Gain  Gain=1/(2*pi)
  Gain1 : Gain  Gain=2*pi
  IC : InitialCondition  Value=0
  Logical Operator : Logic  Operator=OR  AllPortsSameDT=off  OutDataTypeStr=boolean
  Rounding Function : Rounding
  Sum1 : Sum  Inputs=|+-
  θ : Outport
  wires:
  Gain1/1 -> Sum1/2
  Gain/1 -> Rounding Function/1
  IC/1 -> Discrete-Time Integrator/3
  Compare To Constant1/1 -> Logical Operator/2
  Discrete-Time Integrator/State -> Compare To Constant1/1, Sum1/1, Gain/1, Compare To Constant/1
  Compare To Constant/1 -> Logical Operator/1
  Logical Operator/1 -> Discrete-Time Integrator/2
  Sum1/1 -> IC/1
  Rounding Function/1 -> Gain1/1
  ω/1 -> Discrete-Time Integrator/1
  Discrete-Time Integrator/1 -> θ/1

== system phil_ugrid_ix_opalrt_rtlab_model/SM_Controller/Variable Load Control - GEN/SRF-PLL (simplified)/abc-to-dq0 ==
  note: q = -al*sin(wt) + be*cos(wt)
  note: d = al*cos(wt) + be*sin(wt)
  abc : Inport  PortDimensions=3
  wt : Inport  Port=2  PortDimensions=1
  Demux4 : Demux  Outputs=[2 1]
  Fcn : Fcn  Expr=u[1]*cos(u[3]) + u[2]*sin(u[3])
  Fcn1 : Fcn  Expr=-u[1]*sin(u[3]) + u[2]*cos(u[3])
  Gain1 : Gain  Gain=2/3  SaturateOnIntegerOverflow=on
  Gain3 : Gain  Gain="[ 1   -1/2   -1/2; 0   sqrt(3)/2   -sqrt(3)/2; 1/2  1/2  1/2 ]"  Multiplication=Matrix(K*u) (u vector)  SaturateOnIntegerOverflow=on
  Mux : Mux  Inputs=[2 1]
  Mux1 : Mux  Inputs=2
  Mux2 : Mux  Inputs=[2 1]
  Mux3 : Mux  Inputs=[2 1]
  dq0 : Outport
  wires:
  Gain1/1 -> Demux4/1
  abc/1 -> Gain3/1
  Demux4/2 -> Mux/2
  Fcn1/1 -> Mux1/2
  Demux4/1 -> Mux3/1, Mux2/1
  Fcn/1 -> Mux1/1
  Mux2/1 -> Fcn/1
  Mux3/1 -> Fcn1/1
  wt/1 -> Mux2/2, Mux3/2
  Mux/1 -> dq0/1
  Mux1/1 -> Mux/1
  Gain3/1 -> Gain1/1

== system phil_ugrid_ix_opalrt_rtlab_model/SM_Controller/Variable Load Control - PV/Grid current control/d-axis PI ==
  e : Inport
  Kp : Inport  Port=2
  Ki : Inport  Port=3
  reset : Inport  Port=4
  IOut : Product  DisableCoverage=on
  Integrator : DiscreteIntegrator  ExternalReset=level  SampleTime=-1  ICPrevOutput=DiscIntNeverNeededParam  ICPrevScaledInput=DiscIntNeverNeededParam
  POut : Product
  Sum1 : Sum  Inputs=|++
  y : Outport  InitialOutput=0
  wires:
  Integrator/1 -> Sum1/1
  POut/1 -> Sum1/2
  IOut/1 -> Integrator/1
  reset/1 -> Integrator/2
  Kp/1 -> POut/2
  Ki/1 -> IOut/2
  Sum1/1 -> y/1
  e/1 -> IOut/1, POut/1

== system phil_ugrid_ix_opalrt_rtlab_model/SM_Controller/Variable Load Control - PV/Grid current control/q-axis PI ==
  e : Inport
  Kp : Inport  Port=2
  Ki : Inport  Port=3
  reset : Inport  Port=4
  IOut : Product  DisableCoverage=on
  Integrator : DiscreteIntegrator  ExternalReset=level  SampleTime=-1  ICPrevOutput=DiscIntNeverNeededParam  ICPrevScaledInput=DiscIntNeverNeededParam
  POut : Product
  Sum1 : Sum  Inputs=|++
  y : Outport  InitialOutput=0
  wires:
  e/1 -> POut/1, IOut/1
  Sum1/1 -> y/1
  Ki/1 -> IOut/2
  Kp/1 -> POut/2
  reset/1 -> Integrator/2
  IOut/1 -> Integrator/1
  POut/1 -> Sum1/2
  Integrator/1 -> Sum1/1

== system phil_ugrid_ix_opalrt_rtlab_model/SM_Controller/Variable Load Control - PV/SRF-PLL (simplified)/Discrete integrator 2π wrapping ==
  ω : Inport
  Compare To Constant : simulink/Logic and Bit Operations/Compare To Constant  relop=<  const=0  OutDataTypeStr=boolean
  Compare To Constant1 : simulink/Logic and Bit Operations/Compare To Constant  relop=>=  const=2*pi  OutDataTypeStr=boolean
  Discrete-Time Integrator : DiscreteIntegrator  ExternalReset=sampled level  InitialConditionSource=external  SampleTime=-1  ShowStatePort=on  ICPrevOutput=DiscIntNeverNeededParam  ICPrevScaledInput=DiscIntNeverNeededParam
  Gain : Gain  Gain=1/(2*pi)
  Gain1 : Gain  Gain=2*pi
  IC : InitialCondition  Value=0
  Logical Operator : Logic  Operator=OR  AllPortsSameDT=off  OutDataTypeStr=boolean
  Rounding Function : Rounding
  Sum1 : Sum  Inputs=|+-
  θ : Outport
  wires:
  Discrete-Time Integrator/1 -> θ/1
  ω/1 -> Discrete-Time Integrator/1
  Rounding Function/1 -> Gain1/1
  Sum1/1 -> IC/1
  Logical Operator/1 -> Discrete-Time Integrator/2
  Compare To Constant/1 -> Logical Operator/1
  Discrete-Time Integrator/State -> Compare To Constant/1, Gain/1, Sum1/1, Compare To Constant1/1
  Compare To Constant1/1 -> Logical Operator/2
  IC/1 -> Discrete-Time Integrator/3
  Gain/1 -> Rounding Function/1
  Gain1/1 -> Sum1/2

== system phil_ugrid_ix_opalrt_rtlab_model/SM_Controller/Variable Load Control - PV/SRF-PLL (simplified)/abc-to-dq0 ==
  note: d = al*cos(wt) + be*sin(wt)
  note: q = -al*sin(wt) + be*cos(wt)
  abc : Inport  PortDimensions=3
  wt : Inport  Port=2  PortDimensions=1
  Demux4 : Demux  Outputs=[2 1]
  Fcn : Fcn  Expr=u[1]*cos(u[3]) + u[2]*sin(u[3])
  Fcn1 : Fcn  Expr=-u[1]*sin(u[3]) + u[2]*cos(u[3])
  Gain1 : Gain  Gain=2/3  SaturateOnIntegerOverflow=on
  Gain3 : Gain  Gain="[ 1   -1/2   -1/2; 0   sqrt(3)/2   -sqrt(3)/2; 1/2  1/2  1/2 ]"  Multiplication=Matrix(K*u) (u vector)  SaturateOnIntegerOverflow=on
  Mux : Mux  Inputs=[2 1]
  Mux1 : Mux  Inputs=2
  Mux2 : Mux  Inputs=[2 1]
  Mux3 : Mux  Inputs=[2 1]
  dq0 : Outport
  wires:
  Gain3/1 -> Gain1/1
  Mux1/1 -> Mux/1
  Mux/1 -> dq0/1
  wt/1 -> Mux3/2, Mux2/2
  Mux3/1 -> Fcn1/1
  Mux2/1 -> Fcn/1
  Fcn/1 -> Mux1/1
  Demux4/1 -> Mux2/1, Mux3/1
  Fcn1/1 -> Mux1/2
  Demux4/2 -> Mux/2
  abc/1 -> Gain3/1
  Gain1/1 -> Demux4/1
